(* Logix 5000 AddOnInstructionDefinition export AMCI_NXFE2_Preset_Position; software revision 20.03 *)

ADD_ON_INSTRUCTION AMCI_NXFE2_Preset_Position   (* revision 1.0, vendor AMCI *)
VAR_INPUT
   Target_Position : DINT; {required}
END_VAR
VAR_IN_OUT
   NXFE2_output_data : _000A:NXFE2_0986AEB4:O:0; {required}
END_VAR
VAR
   command_data_block : INT[10];
        [0]   // Command Bits MSW
        [1]   // Command Bits LSW
        [2]   // Upper Target Position
        [3]   // Lower Target Position
        [4]   // Upper Programmed Speed
        [5]   // Lower Programmed Speed
END_VAR

ROUTINE Logic   (* ladder *)
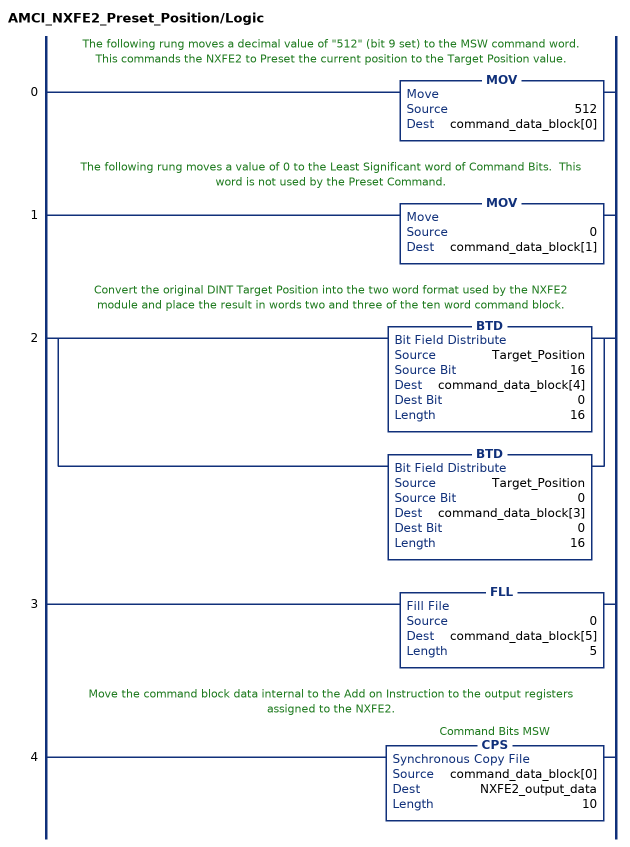
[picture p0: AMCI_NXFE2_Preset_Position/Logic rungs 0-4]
   // The following rung moves a decimal value of "512" (bit 9 set) to the MSW command word.  This commands the NXFE2 to Preset the current position to the Target Position value.
   0: MOV(512,command_data_block[0]);
   // The following rung moves a value of 0 to the Least Significant word of Command Bits.  This word is not used by the Preset Command.
   1: MOV(0,command_data_block[1]);
   // Convert the original DINT Target Position into the two word format used by the NXFE2 module and place the result in words two and three of the ten word command block.
   2: [BTD(Target_Position,16,command_data_block[4],0,16) ,BTD(Target_Position,0,command_data_block[3],0,16) ];
   3: FLL(0,command_data_block[5],5);
   // Move the command block data internal to the Add on Instruction to the output registers assigned to the NXFE2.
   4: CPS(command_data_block[0],NXFE2_output_data,10);
END_ROUTINE
END_ADD_ON_INSTRUCTION
